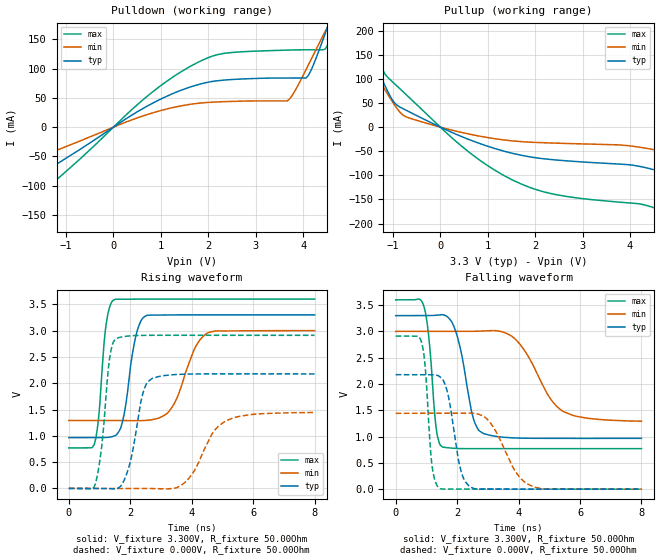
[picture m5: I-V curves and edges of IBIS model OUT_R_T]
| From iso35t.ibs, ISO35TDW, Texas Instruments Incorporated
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|   OUT_R_T  model for ISO35T
[Model]   OUT_R_T
Model_type   Output
| Signals   R
Vmeas = 1.65V
Cref  = 15pF   |Timing specification test load capacitance value
Vref  = 0   |Timing specification test load voltage; GND
| variable   typ   min   max
|R_average   (Slow PVT)   (Nom PVT)   (Fast PVT)
C_comp   2.0200262pF   2.01112935pF   2.0220429pF
|R High state   (Slow PVT)   (typ PVT)   (Fast PVT)
|C_comp   2.0641253pF   2.0560285pF   2.0786956pF
|R Low state   (typ PVT)   (Fast PVT)   (Slow PVT)
|C_comp   1.9662302pF   1.9653902pF   1.9759271pF
[Model Spec]
Vmeas   1.65V   1.5V   1.8V
|   typ   min   max
[Temperature Range]   27.0   85   -40
[Voltage range]   3.3V   3.0V   3.6V
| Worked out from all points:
|   slope of the pulldown table from 0 to 0.495 V, typ, clamps not added: 19.2 ohm
|   slope of the pullup table from 0 to 0.495 V, typ, clamps not added: 23.2 ohm
|   falling waveform, V_fixture 3.300V, R_fixture 50.00Ohm: 20-80 % time 449ps typ, 981ps min, 234ps max; typ from 3.3 V to 0.966 V
|   rising waveform, V_fixture 3.300V, R_fixture 50.00Ohm: 20-80 % time 350ps typ, 647ps min, 227ps max; typ from 0.966 V to 3.3 V
|   rising waveform, V_fixture 0.000V, R_fixture 50.00Ohm: 20-80 % time 413ps typ, 787ps min, 274ps max; typ from 0 V to 2.18 V
|   falling waveform, V_fixture 0.000V, R_fixture 50.00Ohm: 20-80 % time 363ps typ, 751ps min, 197ps max; typ from 2.18 V to 0 V
[Pulldown]
|   Voltage   I(typ)   I(min)   I(max)
-3.3V     -159.9mA   -103.8mA   -221.6mA
-2.405V   -120.4mA   -77.09mA   -168.4mA
-1.111V   -58.78mA   -36.78mA   -83.57mA
729.6mV   36.71mA    21.93mA    53.92mA
1.973V    76.39mA    42.08mA    117.9mA
2.471V    81.23mA    43.89mA    127.3mA
3.665V    83.91mA    44.86mA    131.6mA
4.113V    88.74mA    106.6mA    132.1mA
4.411V    147.9mA    155mA      132.2mA
4.511V    170.1mA    170.7mA    139.4mA
4.66V     203.7mA    193.7mA    179.9mA
6.6V      531.9mA    389.9mA    734.1mA
[Pullup]
|   Voltage   I(typ)   I(min)   I(max)
-3.3V     456.3mA    336.6mA    659mA
-2.007V   264.5mA    206.5mA    359mA
-1.758V   214.2mA    171mA      283.2mA
-1.559V   171.6mA    140.6mA    220mA
-1.211V   95.13mA    84.57mA    117.5mA
-912.1mV  45.49mA    38.54mA    85.14mA
-663.3mV  32.15mA    19.21mA    62.15mA
580.4mV   -24.75mA   -13.81mA   -49.92mA
1.725V    -58.69mA   -30.21mA   -118.7mA
4.262V    -82.61mA   -42.62mA   -160.4mA
5.555V    -119.9mA   -68.73mA   -209.4mA
6.6V      -156.8mA   -94.42mA   -257.4mA
[Ramp]
R_load = 50.00Ohm
|   typ   min   max
dV/dt_r   1.306V/412.754ps 865.587mV/787.211ps   1.746V/274.333ps
dV/dt_f   1.400V/448.889ps   1.025V/981.004ps   1.698V/233.594ps
[Falling Waveform]
V_fixture = 3.300V
V_fixture_min = 3.000V
V_fixture_max = 3.600V
R_fixture = 50.00Ohm
|   Time   V(typ)   V(min)   V(max)
0s        3.3V       3V         3.6V
910ps     3.3V       3V         3.492V
1.32ns    3.308V     3V         1.148V
1.52ns    3.318V     3V         803.1mV
1.95ns    3.006V     3V         775.1mV
2.5ns     1.403V     3.001V     769.6mV
2.82ns    1.07V      3.008V     769.7mV
3.91ns    973.4mV    2.842V     770.2mV
5.45ns    965mV      1.48V      770.3mV
8ns       966mV      1.292V     770.3mV
[Rising Waveform]
V_fixture = 3.300V
V_fixture_min = 3.000V
V_fixture_max = 3.600V
R_fixture = 50.00Ohm
|   Time   V(typ)   V(min)   V(max)
0s        966mV      1.292V     770.3mV
840ps     965.5mV    1.292V     860.8mV
1.2ns     966.8mV    1.292V     3.055V
1.45ns    991.6mV    1.292V     3.581V
1.73ns    1.229V     1.291V     3.596V
2.16ns    2.841V     1.288V     3.599V
2.5ns     3.28V      1.293V     3.6V
3.32ns    3.298V     1.51V      3.6V
4.51ns    3.3V       2.953V     3.6V
8ns       3.3V       3V         3.6V
[Rising Waveform]
V_fixture = 0.000V
V_fixture_min = 0.000V
V_fixture_max = 0.000V
R_fixture = 50.00Ohm
|   Time   V(typ)   V(min)   V(max)
0s        28.4uV     33.36uV    23.08uV
860ps     332.1uV    127.7uV    80.51mV
1.07ns    -265.4uV   147.9uV    794mV
1.33ns    -5.271mV   116.2uV    2.48V
1.54ns    -9.69mV    103.6uV    2.851V
1.92ns    339.7mV    264.9uV    2.896V
2.7ns     2.085V     -2.339mV   2.911V
3.79ns    2.173V     120.6mV    2.911V
5.15ns    2.178V     1.294V     2.911V
8ns       2.177V     1.443V     2.911V
[Falling Waveform]
V_fixture = 0.000V
V_fixture_min = 0.000V
V_fixture_max = 0.000V
R_fixture = 50.00Ohm
|   Time   V(typ)   V(min)   V(max)
0s        2.177V     1.443V     2.911V
840ps     2.177V     1.443V     2.8V
970ps     2.178V     1.443V     2.256V
1.18ns    2.178V     1.443V     458.6mV
1.43ns    2.141V     1.443V     14.39mV
1.7ns     1.809V     1.443V     2.367mV
2.12ns    361.2mV    1.445V     163.7uV
2.43ns    41.51mV    1.446V     -80.13uV
4.43ns    16.15uV    59.79mV    28.66uV
8ns       28.4uV     33.36uV    23.08uV
